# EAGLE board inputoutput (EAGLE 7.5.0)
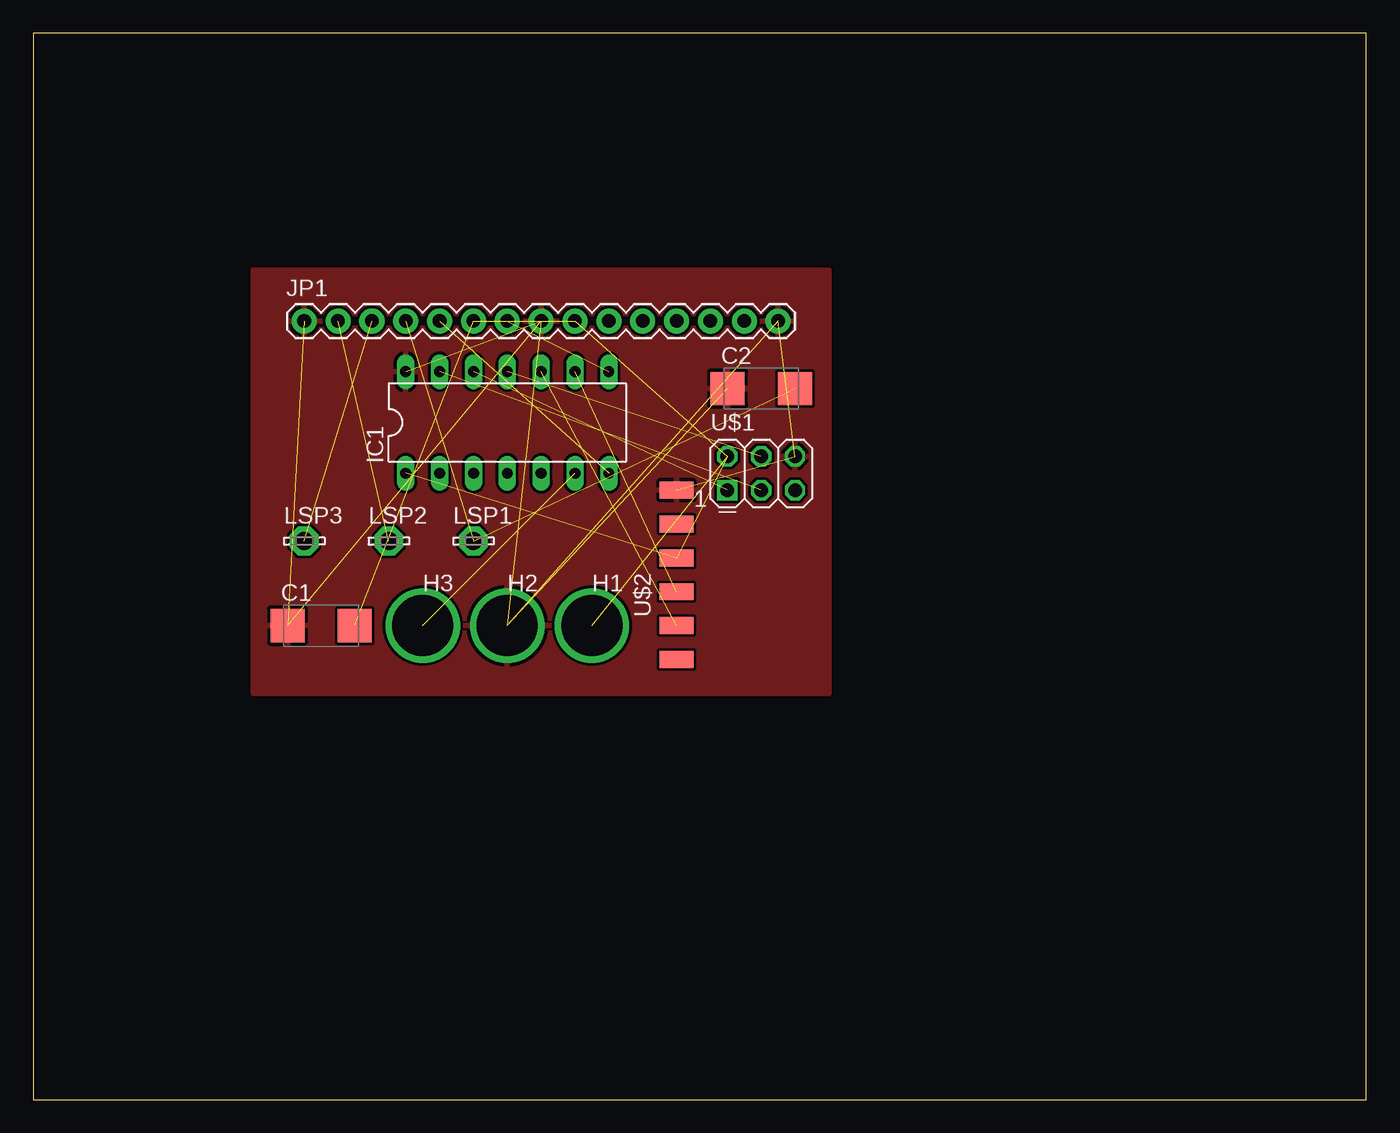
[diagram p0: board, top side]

Size 100 x 80 mm. Coordinates in mm from the lower left corner, seen from the top.
Outline: 0,0 100,0 100,80 0,80 0,0
Copper layers (1*16): Top 0.035mm / dielectric 1.5mm / Bottom 0.035mm
Design rules "default": minimum track width 10mil, minimum drill 24mil, track to track 8mil, track to pad 8mil, pad to pad 8mil, via to via 8mil, smd to smd 8mil, copper to edge 40mil, drill to drill 8mil, minimum pad ring 10mil, minimum via ring 8mil, stop-mask expansion 4mil, vias tented up to drill 0mil, thermal gap 10mil

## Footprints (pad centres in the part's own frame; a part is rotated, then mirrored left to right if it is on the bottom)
C/6032-28R = smd 2.55 x 2.5: + 2.525,0; - -2.525,0
PAD_0.1800 = drill 4.572 pad 4.572: 1 0,0
DIL14 = drill 0.813 long: 1 -7.62,-3.81; 2 -5.08,-3.81; 3 -2.54,-3.81; 4 0,-3.81; 5 2.54,-3.81; 6 5.08,-3.81; 7 7.62,-3.81; 8 7.62,3.81; 9 5.08,3.81; 10 2.54,3.81; 11 0,3.81; 12 -2.54,3.81; 13 -5.08,3.81; 14 -7.62,3.81
1X15 = drill 1.016 pad 1.88: 1 0,0; 2 2.54,0; 3 5.08,0; 4 7.62,0; 5 10.16,0; 6 12.7,0; 7 15.24,0; 8 17.78,0; 9 20.32,0; 10 22.86,0; 11 25.4,0; 12 27.94,0; 13 30.48,0; 14 33.02,0; 15 35.56,0
LSP13 = drill 1.321 pad 2.159 octagon: MP 0,0
2X03 = drill 1.016 square: 1 -2.54,-1.27 | drill 1.016 octagon: 2 -2.54,1.27; 3 0,-1.27; 4 0,1.27; 5 2.54,-1.27; 6 2.54,1.27
1X06SMD = smd 2.54 x 1.27: 1 0,6.35; 2 0,3.81; 3 0,1.27; 4 0,-1.27; 5 0,-3.81; 6 0,-6.35

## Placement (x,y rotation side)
C1  2.2u  [C/6032-28R]  21.59,35.56 0 top
C2  2.2u  [C/6032-28R]  54.61,53.34 0 top
H1  [PAD_0.1800]  41.91,35.56 0 top
H2  [PAD_0.1800]  35.56,35.56 0 top
H3  [PAD_0.1800]  29.21,35.56 0 top
IC1  ATTINY44-PU  [DIL14]  35.56,50.8 0 top
JP1  M15  [1X15]  20.32,58.42 0 top
LSP1  LSP13  [LSP13]  33.02,41.91 0 top
LSP2  LSP13  [LSP13]  26.67,41.91 0 top
LSP3  LSP13  [LSP13]  20.32,41.91 0 top
U$1  AVRISP  [2X03]  54.61,46.99 0 top
U$2  FTDI-SMD-HEADER  [1X06SMD]  48.26,39.37 0 top

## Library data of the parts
C1 C2 = rcl
H1-H3 = special-drill
IC1 U$1 U$2 = fab
JP1 = SparkFun
LSP1-LSP3 = solpad

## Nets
+5V: C1.+ H1.1 IC1.1 JP1.6 JP1.9 U$1.2 U$2.3
ENB: JP1.11
GND: C1.- C2.- H2.1 IC1.14 JP1.1 JP1.8 JP1.15 U$1.6 U$2.1
IN2: IC1.8 JP1.7
IN3: JP1.10
IN4: JP1.12
N$1: IC1.7 JP1.5
N$2: C2.+ JP1.4 LSP1.MP
N$3: H3.1 IC1.6
N$4: U$1.5
N$5: IC1.13 U$1.3
N$6: IC1.12 U$1.1
N$7: IC1.11 U$1.4
N$8: IC1.9 U$2.4
N$9: IC1.10 U$2.5
OUT1: JP1.2 LSP2.MP
OUT2: JP1.3 LSP3.MP
OUT3: JP1.13
OUT4: JP1.14

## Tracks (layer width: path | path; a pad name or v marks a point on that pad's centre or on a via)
+5V  (6 unrouted)
GND  (8 unrouted)
  pour Top: 16.51,62.23 59.69,62.23 59.69,59.69 59.69,30.48 16.51,30.48
IN2  (1 unrouted)
N$1  (1 unrouted)
N$2  (2 unrouted)
N$3  (1 unrouted)
N$5  (1 unrouted)
N$6  (1 unrouted)
N$7  (1 unrouted)
N$8  (1 unrouted)
N$9  (1 unrouted)
OUT1  (1 unrouted)
OUT2  (1 unrouted)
